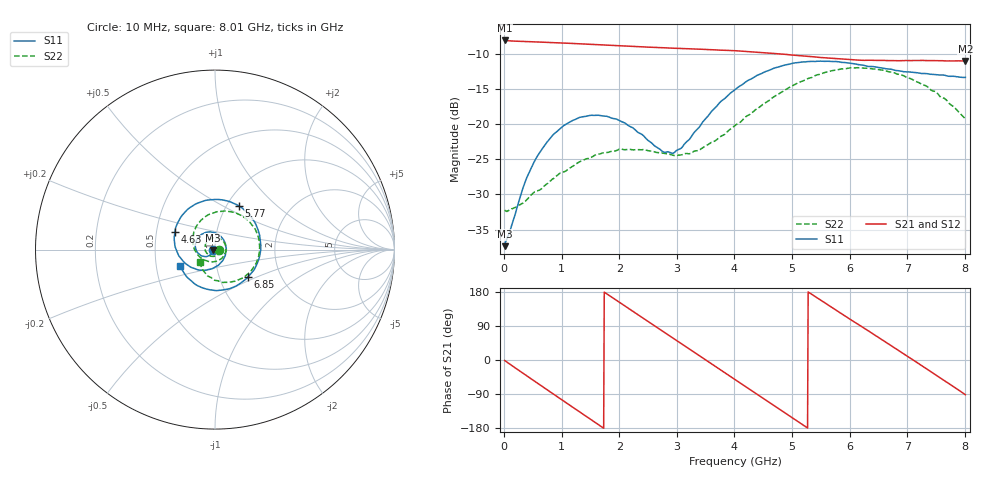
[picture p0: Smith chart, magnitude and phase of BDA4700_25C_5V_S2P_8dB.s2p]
!Agilent Technologies,E5071B,MY42404982,A.09.10
!Date: Mon Oct 20 13:30:00 2025
!Data & Calibration Information:
!Freq	S11:SOLT2(ON)	S21:SOLT2(ON)	S12:SOLT2(ON)	S22:SOLT2(ON)
# Hz S RI R 50
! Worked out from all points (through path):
!   801 points, 10 MHz to 8.01 GHz, reference 50 ohm
!   highest |S21| = -8.12 dB at 10 MHz (marker M1); lowest = -11.0 dB at 8.01 GHz (marker M2)
!   group delay of S21, straight-line fit = 281 ps
!   lowest |S11| = -37.3 dB at 10 MHz (marker M3), VSWR 1.03, Z = 48.7 - j0.168 ohm
!   |S11| at or under -10 dB: start of sweep to end of sweep
!   |S22| runs from -32.4 to -12.0 dB; largest |S21 - S12| = 0.0029
!   S11 on the Smith chart (normalised r, x): 10 MHz: 0.97, -0.00; 4.63 GHz: 0.62, +0.13; 5.77 GHz: 1.14, +0.60; 6.85 GHz: 1.36, -0.45; 8.01 GHz: 0.66, -0.12
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1e7  -0.0135 -0.00173  0.3926 -0.00858  0.3924 -0.00884  0.0245 -0.00137
3.6e8  -0.0259 -0.0281  0.3037 -0.2383  0.3036 -0.2388  0.0196 -0.02
5.8e8  -0.0452 -0.0384  0.1853 -0.3351  0.1852 -0.3355  0.00958 -0.0322
9.5e8  -0.0869 -0.0268  -0.0623 -0.3724  -0.0622 -0.3723  -0.0251 -0.0364
1.35e9  -0.1101 0.0233  -0.2879 -0.2344  -0.2882 -0.2345  -0.0547 -0.00266
1.93e9  -0.0541 0.0947  -0.3386 0.1266  -0.3387 0.1268  -0.0214 0.0608
2.32e9  0.013 0.0866  -0.1761 0.308  -0.1762 0.3081  0.0318 0.0577
2.68e9  0.0566 0.0367  0.041 0.3474  0.0409 0.3473  0.0608 0.0148
2.95e9  0.06 -0.0179  0.1939 0.2865  0.1937 0.2861  0.055 -0.0234
3.37e9  0.00927 -0.0925  0.3314 0.079  0.3319 0.0789  0.0079 -0.0643
3.68e9  -0.0655 -0.1149  0.3198 -0.1042  0.3199 -0.1051  -0.0422 -0.064
4.01e9  -0.1531 -0.0859  0.2057 -0.2606  0.2059 -0.2602  -0.0912 -0.0344
4.32e9  -0.2121 -0.00914  0.0382 -0.3233  0.038 -0.3239  -0.12 0.0211
4.63e9  -0.2233 0.0964  -0.1342 -0.2889  -0.134 -0.2892  -0.1188 0.0928
5e9  -0.1593 0.2173  -0.2739 -0.1437  -0.2745 -0.1441  -0.0653 0.1748
5.35e9  -0.0352 0.2767  -0.2984 0.0391  -0.2986 0.0383  0.0334 0.2124
5.77e9  0.1349 0.2432  -0.1912 0.2201  -0.1909 0.2204  0.1662 0.1765
6.21e9  0.2446 0.0962  0.00938 0.2839  0.0118 0.2842  0.2461 0.0481
6.68e9  0.2266 -0.0969  0.2104 0.1885  0.2109 0.1884  0.2112 -0.1036
6.85e9  0.1832 -0.1541  0.255 0.1198  0.2557 0.1187  0.1737 -0.1446
7.37e9  -0.008 -0.227  0.2524 -0.1273  0.2524 -0.1276  0.0294 -0.1794
8.01e9  -0.1954 -0.0892  -0.00778 -0.2805  -0.0072 -0.2808  -0.0862 -0.0666
